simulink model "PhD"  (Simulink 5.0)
settings: Solver=ode4  StartTime=0.0  StopTime=2.5  FixedStep=0.0002  RelTol=1e-3
libraries: simulink x1

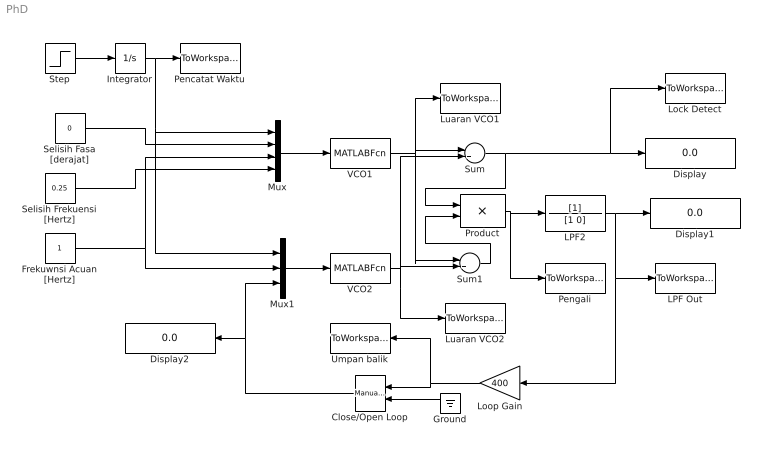
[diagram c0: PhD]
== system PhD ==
  Close/Open Loop : simulink/Signal Routing/Manual Switch  Orientation=left  sw=1  action=0
  Display : Display
  Display1 : Display
  Display2 : Display
  Frekuwnsi Acuan [Hertz] : Constant
  Ground : Ground  Orientation=left
  Integrator : Integrator
  LPF Out : ToWorkspace  VariableName=lpfout  SampleTime=-1  SaveFormat=Array
  LPF2 : TransferFcn  Denominator=[1 0]
  Lock Detect : ToWorkspace  VariableName=lockdetect  SampleTime=-1  SaveFormat=Array
  Loop Gain : Gain  Orientation=left  Gain=400
  Luaran VCO1 : ToWorkspace  VariableName=outvco1  SampleTime=-1  SaveFormat=Array
  Luaran VCO2 : ToWorkspace  VariableName=outvco2  SampleTime=-1  SaveFormat=Array
  Mux : Mux
  Mux1 : Mux  Inputs=3
  Pencatat Waktu : ToWorkspace  VariableName=time  SampleTime=-1  SaveFormat=Array
  Pengali : ToWorkspace  VariableName=outprod  SampleTime=-1  SaveFormat=Array
  Product : Product
  Selisih Fasa [derajat] : Constant  Value=0
  Selisih Frekuensi [Hertz] : Constant  Value=0.25
  Step : Step  Time=0  SampleTime=0
  Sum : Sum  Inputs=|+-
  Sum1 : Sum  Inputs=|++
  Umpan balik : ToWorkspace  VariableName=feedback  SampleTime=-1  SaveFormat=Array
  VCO1 : MATLABFcn  MATLABFcn=vco1
  VCO2 : MATLABFcn  MATLABFcn=vco2
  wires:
  Step/1 -> Integrator/1
  Integrator/1 -> Pencatat Waktu/1, Mux/1, Mux1/1
  Frekuwnsi Acuan [Hertz]/1 -> Mux1/2, Mux/3
  Selisih Fasa [derajat]/1 -> Mux/2
  Selisih Frekuensi [Hertz]/1 -> Mux/4
  Mux/1 -> VCO1/1
  Mux1/1 -> VCO2/1
  VCO1/1 -> Sum/1, Luaran VCO1/1, Sum1/1
  VCO2/1 -> Sum/2, Luaran VCO2/1, Sum1/2
  Sum/1 -> Product/1, Display/1, Lock Detect/1
  Product/1 -> LPF2/1, Pengali/1
  LPF2/1 -> Display1/1, Loop Gain/1, LPF Out/1
  Sum1/1 -> Product/2
  Ground/1 -> Close/Open Loop/2
  Loop Gain/1 -> Close/Open Loop/1, Umpan balik/1
  Close/Open Loop/1 -> Mux1/3, Display2/1
